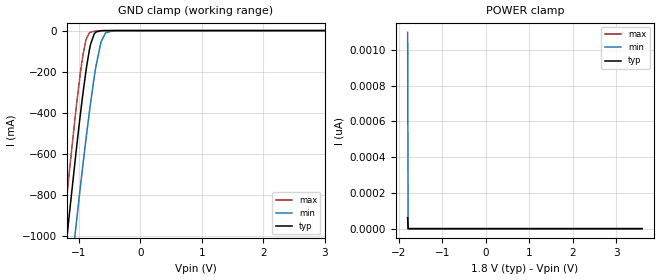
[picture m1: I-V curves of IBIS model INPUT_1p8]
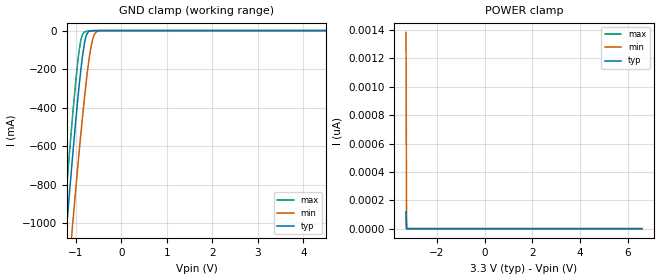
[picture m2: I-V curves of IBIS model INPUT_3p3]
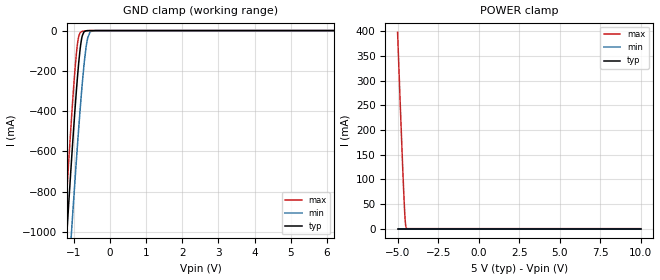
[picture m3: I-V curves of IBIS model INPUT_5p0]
|Texas Instruments Incorporated
|DACx3401 is a signle channel I2C interface, Buffered Voltage Output DAC
|DACx3401 comes in a Tiny 2*2 WSON package
[IBIS Ver] 4.1
[File name] dac53401.ibs
[File Rev] 1.0
[Date] 15/11/2019
[Source]
| Texas Instruments Incorporated.
| 12500 TI Blvd
| Dallas, TX -75243
[Notes] Revision History:
| Rev 1.0: 02/18/2019
| - Initial version of the model
| - Model generated from simulations in TISPICE/SPECTRE
|	Model names with a trailing _1p8 constain model for 1.8V operation.
|	Model names with a trailing _3p3 constain model for 3.3V operation.
|	Model names with a trailing _5p0 constain model for 5.0V operation.
| - C_comp although listed in numerical order of value are
| obtained from varying PVT conditions. For PVT conditions for
| each specific value refer the buffer description under
| respective [Model]. IBIS model user is responsible for using
| appropriate C_comp to simulate for Signal Integrity.
| - Warnings regarding combined Non-monotonicity of various models have been
| reviewed and considered minor and can be ignored.
[Disclaimer]
| This model is designed as an aid for customers of Texas Instruments.
| TI and its licensors and suppliers make no warranties, either expressed
| or implied, with respect to this  model, including the warranties of
| merchantability or fitness for a particular purpose. The model is
| provided solely on an "as is" basis. The entire risk as to its quality
| and performance is with the customer.
| This model is subject to change without notice. Texas Instruments
| Incorporated is not responsible for updating this model.
[Copyright]
(C) Copyright 2018 Texas Instruments Incorporated.All rights reserved.
|  Component DAC53401 8-pin WSON
|  Part # DAC53401
[Component]   dac53401
[Manufacturer]  TI
[Package]   |8-pin WSON
|   typ   min   max
R_pkg   0.05   0.04   0.06
L_pkg   1.0nH   0.8nH   1.2nH
C_pkg   0.2pF   0.16pF   0.24pF
[Pin]   signal_name   model_name   R_pin   L_pin   C_pin
1   A0   INPUT   NA   NA   NA
2   SCL   INPUT   NA   NA   NA
3   SDA   IO_OPENDRAIN   NA   NA   NA
4   CAP   NC   NA   NA   NA
5   AGND   GND   NA   NA   NA
6   VDD   POWER   NA   NA   NA
7   FB   NC   NA   NA   NA
8   VOUT   NC   NA   NA   NA
|   Model Selectors
[Model Selector] IO_OPENDRAIN
OPENDRAIN_1p8  1.8V   digital I/O_open_drain
OPENDRAIN_3p3  3.3V   digital I/O_open_drain
OPENDRAIN_5p0  5.0V   digital I/O_open_drain
[Model Selector] INPUT
INPUT_1p8   1.8V   digital Input
INPUT_3p3   3.3V   digital Input
INPUT_5p0   5.0V   digital Input
| Models and submodels in the file (6): INPUT_1p8 (Input), INPUT_3p3 (Input), INPUT_5p0 (Input), OPENDRAIN_1p8 (I/O_open_drain), OPENDRAIN_3p3 (I/O_open_drain), OPENDRAIN_5p0 (I/O_open_drain)
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|   INPUT_1p8 Model
[Model]   INPUT_1p8
Model_type   Input
Vinl =  0.4
Vinh = 1.62
|   typ   min   max
C_comp   1.651pF   1.620pF   1.681pF
[Voltage Range]   1.8   1.71   1.89
[Temperature Range]   25   125   -40
[Power Clamp Reference]   1.8   1.71   1.89
[GND Clamp Reference]   0   0   0
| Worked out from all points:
|   GND clamp passes 1 mA (typ) near -0.65 V on its own axis
[GND Clamp]
|   Voltage   I(typ)   I(min)   I(max)
-1.8V     -2.802A    -3.099A    -2.651A
-1.433V   -1.696A    -2.028A    -1.51A
-1.195V   -998.9mA   -1.351A    -793.1mA
-1.179V   -952.5mA   -1.305A    -745.6mA
-1.049V   -591.8mA   -948.6mA   -382.1mA
-936mV    -304.3mA   -650.3mA   -118.6mA
-882mV    -185.3mA   -515.6mA   -40.67mA
-817.2mV  -73.14mA   -363.2mA   -8.408mA
-752.4mV  -15.81mA   -225.6mA   -3.254mA
-639mV    -589uA     -52.66mA   -580.8uA
-444.6mV  -4.027uA   -369.8uA   -3.003uA
3.6V      0A         0A         0A
[POWER Clamp]
|   Voltage   I(typ)   I(min)   I(max)
-1.8V     61.34pA    1.099nA    61.94pA
-1.789V   0A         0A         0A
-1.784V   0A         0A         0A
3.6V      0A         0A         0A
|   INPUT_3p3 Model
[Model]   INPUT_3p3
Model_type   Input
Vinl = 0.4
Vinh = 1.62
|   typ   min   max
C_comp   1.492pF   1.464pF   1.512pF
[Voltage Range]   3.3   3   3.6
[Temperature Range]   25   125   -40
[Power Clamp Reference]   3.3   3   3.6
[GND Clamp Reference]   0   0   0
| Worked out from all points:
|   GND clamp passes 1 mA (typ) near -0.66 V on its own axis
[GND Clamp]
|   Voltage   I(typ)   I(min)   I(max)
-3.3V     -7.413A    -7.565A    -7.396A
-1.34V    -1.42A     -1.761A    -1.226A
-1.261V   -1.188A    -1.535A    -987.2mA
-1.211V   -1.045A    -1.396A    -839.9mA
-1.073V   -654.3mA   -1.011A    -443.9mA
-933.9mV  -299.4mA   -644.9mA   -114.7mA
-884.4mV  -190.3mA   -521.4mA   -43.06mA
-805.2mV  -57.92mA   -336.5mA   -6.729mA
-745.8mV  -13.07mA   -212.7mA   -3mA
-646.8mV  -722.6uA   -60.46mA   -673.7uA
-498.3mV  -18.34uA   -1.697mA   -18.68uA
6.6V      0A         0A         0A
[POWER Clamp]
|   Voltage   I(typ)   I(min)   I(max)
-3.3V     115.3pA    1.383nA    120.2pA
-3.28V    0A         0A         0A
-3.27V    0A         0A         0A
6.6V      0A         0A         0A
|   INPUT_5p0 Model
[Model]   INPUT_5p0
Model_type   Input
Vinl = 0.4
Vinh = 1.62
|   typ   min   max
C_comp   1.373pF   1.354pF   1.392pF
[Voltage Range]   5   4.5   5.5
[Temperature Range]   25   125   -40
[Power Clamp Reference]   5   4.5   5.5
[GND Clamp Reference]   0   0   0
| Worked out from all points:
|   GND clamp passes 1 mA (typ) near -0.66 V on its own axis
[GND Clamp]
|   Voltage   I(typ)   I(min)   I(max)
-5V       -12.53A    -12.2A     -12.94A
-1.565V   -2.092A    -2.411A    -1.918A
-1.25V    -1.157A    -1.505A    -955.5mA
-1.16V    -898.4mA   -1.252A    -690.3mA
-1.07V    -647.5mA   -1.004A    -437.1mA
-920mV    -267.4mA   -609.8mA   -90.63mA
-860mV    -142.5mA   -462.6mA   -23.4mA
-785mV    -37.12mA   -292.6mA   -4.932mA
-710mV    -4.438mA   -147.8mA   -1.883mA
-620mV    -363.3uA   -36.57mA   -397.1uA
-410mV    -1.355uA   -137.3uA   -776.9nA
10V       0A         0A         0A
[POWER Clamp]
|   Voltage   I(typ)   I(min)   I(max)
-5V       1.401nA    3.976nA    398.1mA
-4.865V   0A         0A         278.4mA
-4.76V    0A         0A         187.4mA
-4.67V    0A         0A         112.7mA
-4.61V    0A         0A         66.4mA
-4.565V   0A         0A         35.84mA
-4.535V   0A         0A         19.34mA
-4.52V    0A         0A         12.91mA
-4.49V    0A         0A         4.525mA
-4.445V   0A         0A         593.7uA
10V       0A         0A         0A
